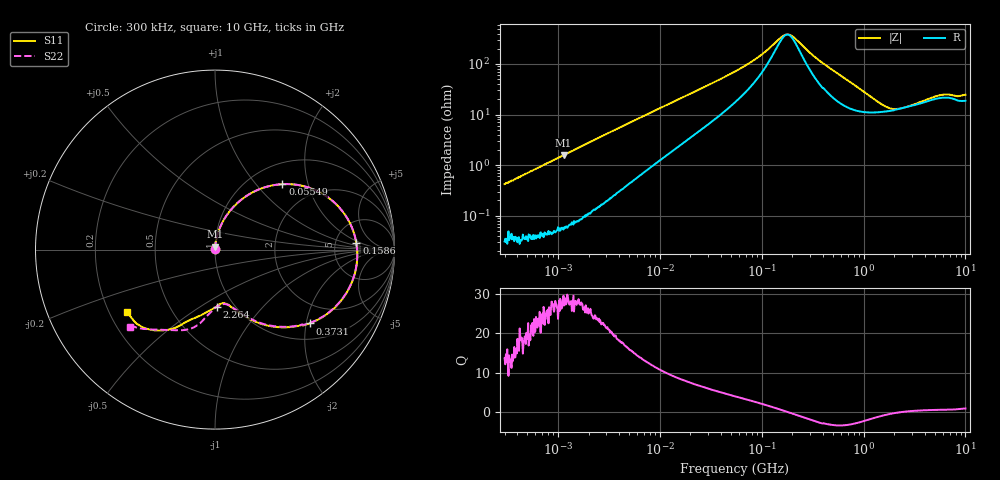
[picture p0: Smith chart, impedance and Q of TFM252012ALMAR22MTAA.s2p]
! S-Parameter Data Generated by TDK Corporation
! Copyright(C) 2019 TDK Corporation.
! All Rights Reserved.
! TDK P/N: TFM252012ALMAR22MTAA (Inductor)
! Property: L=220nH at 1MHz
! Size(LxWxT): 2.5x2x1.2mm
! Model Type: s2p (Touchstone File Format Version 1.0)
! Frequency: DC=Yes Start=0.3MHz Stop=10000MHz 802points Log-sweep
! Model Generated on May 10, 2019
! Port Assignments:
!  1 ---@@@--- 2
! Applicable Conditions:
!  Temperature = 25 degC
!  DC Bias Current = 0 A
!  Small Signal Operation
! Terms and conditions regarding TDK Simulation Models
! (1)This simulation model is being provided solely for informational purposes. Please refer to the specifications of the products in terms of detailed characteristics of such products.
! (2)In no event shall TDK Corporation of any of its subsidiaries be liable for any loss or damage arising, directly or indirectly,
!  From any information contained in this simulation model, including, but not limited to loss or damages arising from any inaccuracies, omissions or errors in connection with such information.
! (3)Any and all copyrights on this simulation model are owned by TDK Corporation.
!  Duplication or redistribution of this simulation model without prior written permission from TDK Corporation is prohibited.
! (4)This simulation model is subject to any modification or change without any prior notice.
! (5)Neither TDK Corporation nor any of its subsidiaries shall make any warranty, express or implied,
!  Including but not limited to the correctness, implied warranties of merchantability and fitness for a particular purpose with respect to this simulation models.
! (6)The use of this simulation model shall be deemed to have consented to the terms and conditions hereof.
# Hz S MA R 50
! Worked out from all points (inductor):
!   801 points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, 300 kHz to 10 GHz, reference 50 ohm
!   read as one part in series: L = 221 nH near 318.3 kHz
!   highest Q = 28.2 at 1.136 MHz (marker M1), where L = 220 nH
!   self-resonance near 179 MHz
!   S11 on the Smith chart (normalised r, x): 300 kHz: 1.00, +0.01; 55.49 MHz: 1.39, +1.39; 158.6 MHz: 8.14, +1.57; 373.1 MHz: 1.41, -2.09; 2.264 GHz: 0.83, -0.59; 10 GHz: 0.27, -0.30
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300000  0.004167 86.2  0.9996 -0.3  0.9994 -0.2  0.004346 89.4
1136463  0.01556 87.0  0.9993 -0.9  0.9994 -0.9  0.01568 87.3
1713600  0.0235 86.4  0.9989 -1.4  0.9988 -1.4  0.02353 86.6
9671944  0.1252 77.4  0.9806 -7.3  0.9807 -7.3  0.1252 77.4
2.567637e7  0.2968 63.6  0.91 -17.5  0.9101 -17.5  0.2967 63.6
5.477226e7  0.5188 44.6  0.736 -31.1  0.7361 -31.1  0.5188 44.6
5.548994e7  0.5231 44.2  0.7315 -31.3  0.7316 -31.3  0.523 44.2
9.444554e7  0.6904 25.3  0.4943 -40.6  0.4944 -40.6  0.6903 25.3
1.585658e8  0.7883 2.6  0.227 -21.2  0.2271 -21.2  0.7881 2.8
1.945824e8  0.7931 -7.0  0.2153 11.0  0.2154 11.0  0.7927 -6.8
3.126428e8  0.7208 -29.8  0.4568 35.9  0.4569 35.9  0.7205 -29.6
3.730642e8  0.6686 -37.9  0.5565 33.1  0.5566 33.1  0.6685 -37.6
5.225392e8  0.5504 -51.6  0.7034 23.8  0.7035 23.8  0.551 -51.0
8.18524e8  0.4055 -66.1  0.8167 10.0  0.8168 10.0  0.4073 -65.3
1.196827e9  0.3269 -74.8  0.8509 -1.2  0.8509 -1.2  0.3303 -74.1
1.767019e9  0.3024 -83.0  0.8482 -12.9  0.8483 -12.9  0.3079 -83.1
2.264206e9  0.3178 -88.2  0.8299 -20.6  0.83 -20.6  0.3235 -89.7
4.865898e9  0.4411 -112.5  0.6982 -48.1  0.6981 -48.1  0.4701 -108.8
6.091595e9  0.4962 -117.8  0.6396 -57.9  0.6397 -58.0  0.5144 -119.4
7.222042e9  0.5573 -126.0  0.5844 -66.7  0.5845 -66.8  0.5739 -129.3
8.434726e9  0.5993 -135.8  0.5457 -74.4  0.5456 -74.4  0.6227 -136.4
1e10  0.5999 -144.4  0.5145 -83.3  0.5145 -83.4  0.6406 -137.7
